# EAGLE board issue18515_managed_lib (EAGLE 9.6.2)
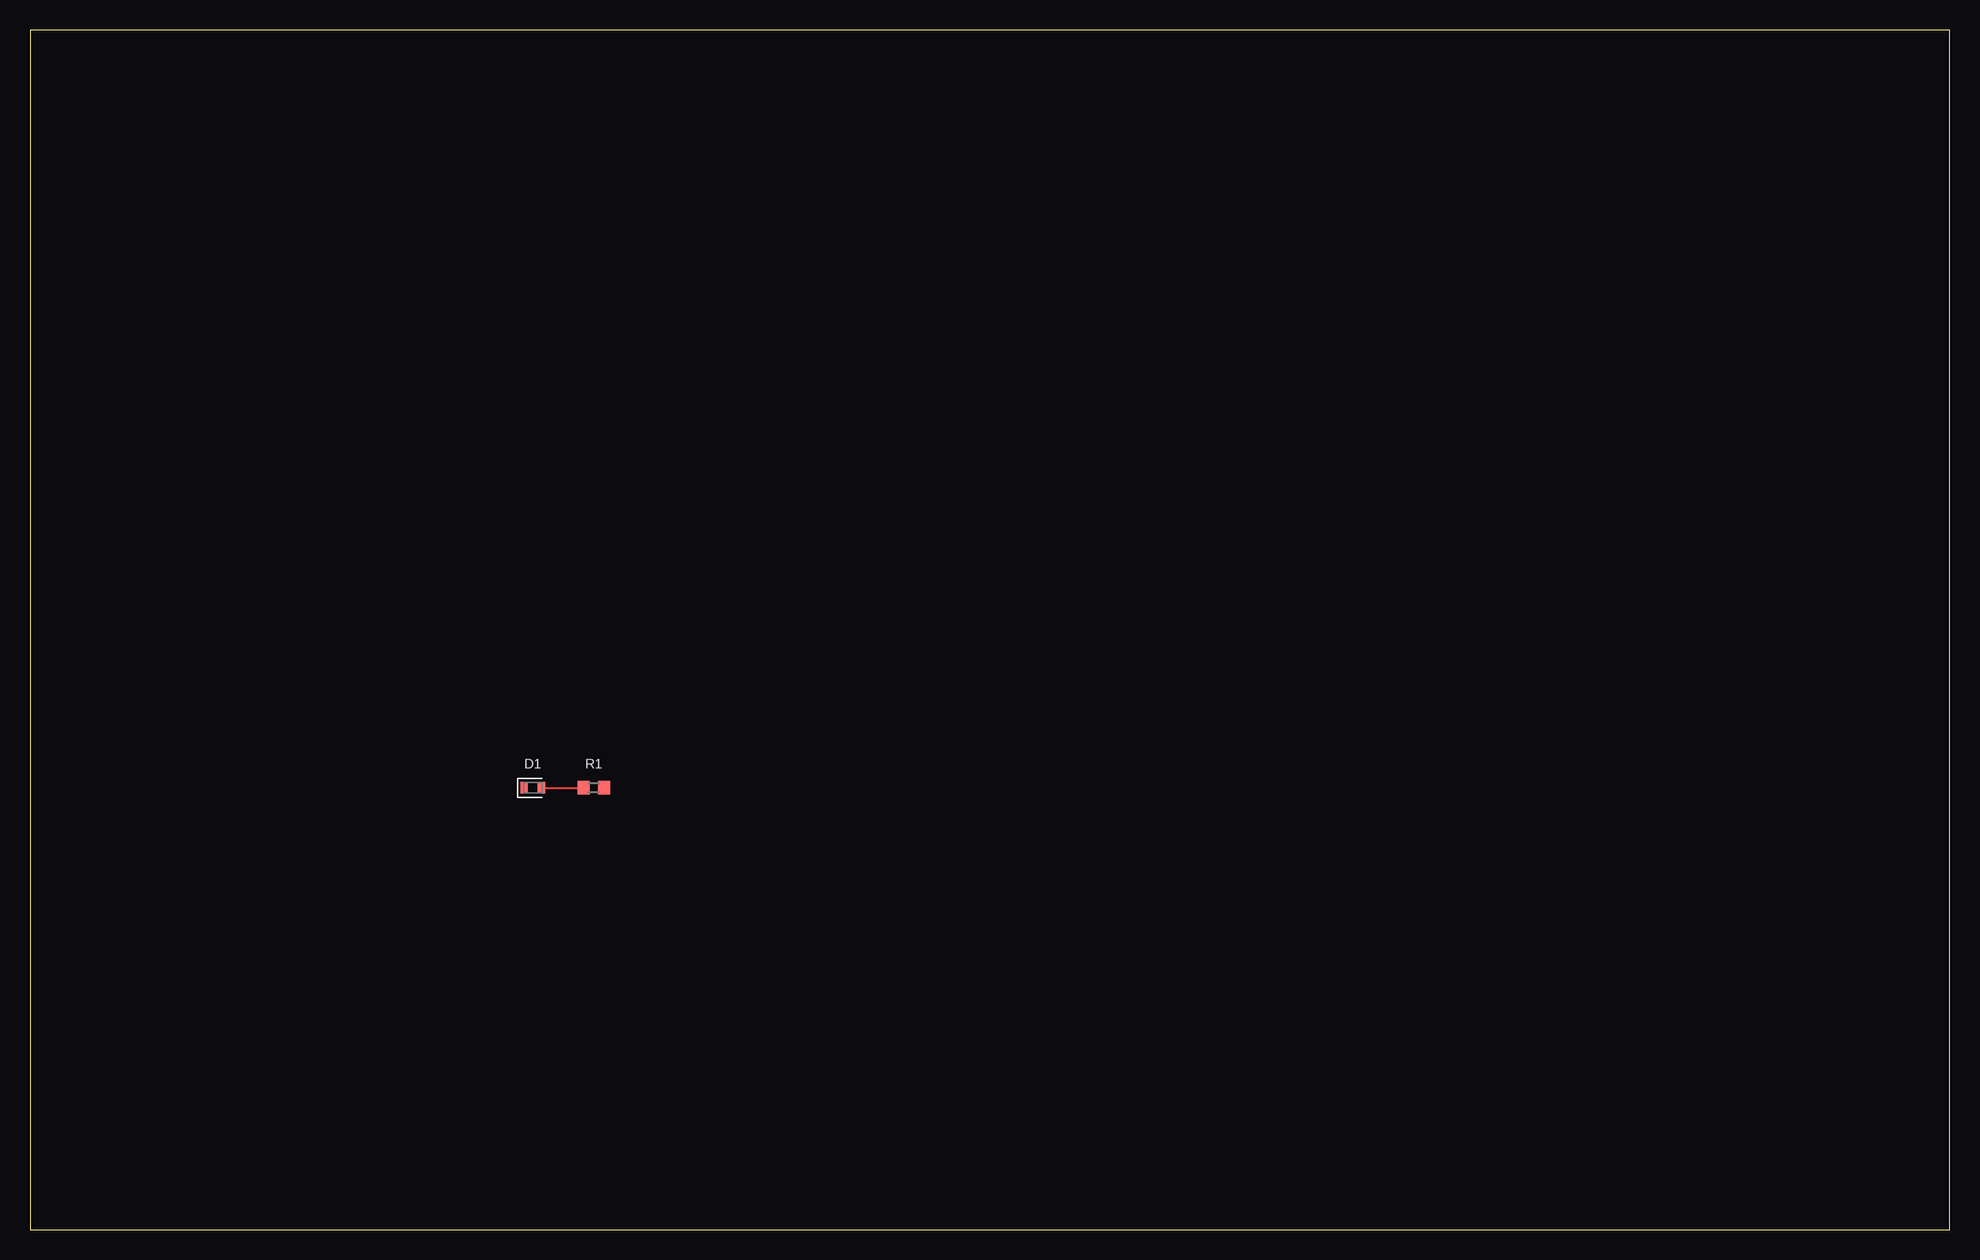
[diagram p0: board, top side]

Size 160 x 100 mm. Coordinates in mm from the lower left corner, seen from the top.
Outline: 0,0 160,0 160,100 0,100 0,0
Copper layers (1*16): Top 0.035mm / dielectric 1.5mm / Bottom 0.035mm
Design rules "default": minimum track width 6mil, minimum drill 0.35mm, track to track 6mil, track to pad 6mil, pad to pad 6mil, via to via 6mil, smd to smd 6mil, copper to edge 40mil, drill to drill 6mil, minimum pad ring 10mil, minimum via ring 8mil, stop-mask expansion 4mil, vias tented up to drill 0mil, thermal gap 10mil

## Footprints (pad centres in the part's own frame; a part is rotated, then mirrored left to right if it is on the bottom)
LED-0603 = smd 0.612 x 0.962: 1 -0.725,0; 2 0.725,0
R0603 = smd 1 x 1.1: 1 -0.85,0; 2 0.85,0

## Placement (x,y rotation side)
D1  CHIP-LED-GREEN  [LED-0603]  41.91,36.83 0 top
R1  [R0603]  46.99,36.83 0 top

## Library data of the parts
D1 = MX_LIB; CURR_RATING: 20mA; GENERIC: Allowed; LCSC_0: C125098; LCSC_2: C125094; LCSC_3: C510025; MFR_0: Lite-on; MFR_2: Lite-on; MFR_3: ROHM; PN_0: LTST-C191KGKT; PN_2: LTST-C190KGKT; PN_3: SML-D12M8WT86; RISK: 1; UNIT_COST: 0.01
R1 = MX_LIB; GENERIC: Allowed; PWR_RATING: 0.1W; RISK: 1; TOLERANCE: 1%; UNIT_COST: 0.02; VTG_RATING: 50V

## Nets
N$1: D1.2 R1.1

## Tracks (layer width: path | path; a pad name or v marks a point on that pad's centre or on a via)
N$1
  Top 0.152: D1.2 R1.1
